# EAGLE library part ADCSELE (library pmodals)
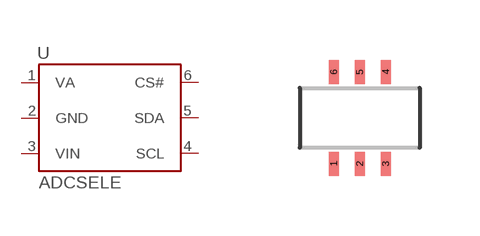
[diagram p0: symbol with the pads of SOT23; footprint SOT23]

Designator prefix -

## ADCSELEA  [SOT23]
1  VA
2  GND
3  VIN
4  SCL
5  SDA
6  CS#

## Footprint SOT23 (pad centres in mm)
smd 0.25 x 0.6: 1 -0.65,-1.15; 2 0,-1.15; 3 0.65,-1.15; 4 0.65,1.15; 5 0,1.15; 6 -0.65,1.15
